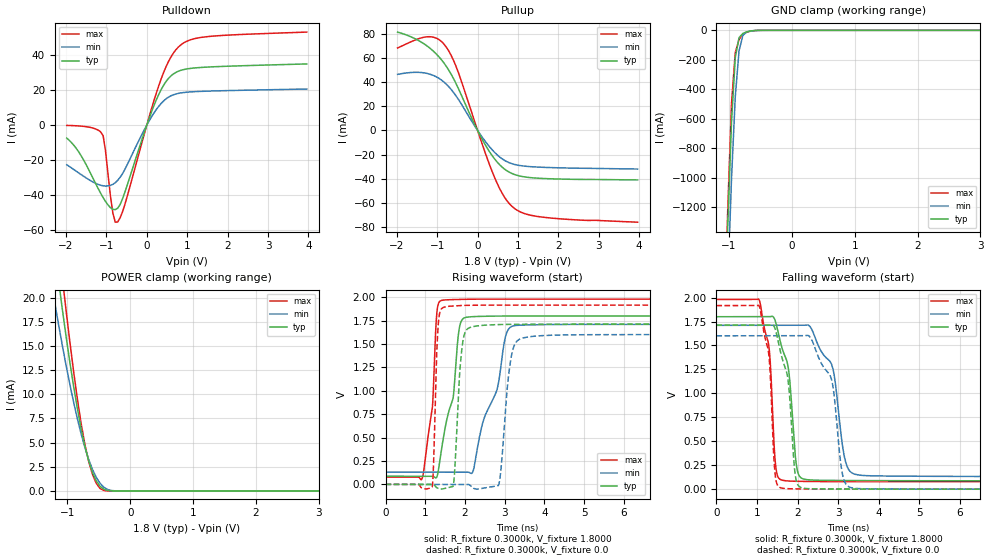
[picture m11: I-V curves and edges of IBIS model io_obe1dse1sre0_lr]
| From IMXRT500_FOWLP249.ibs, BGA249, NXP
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[Model] io_obe1dse1sre0_lr
|   Model io_obe1dse1sre0_lr
| Library cells for typ/min/max conditions are connected as defined below:
|  pad - External Pad
|  ipp_do - Core Input
|  ipp_obe - Output Buffer Enable
|  REFH3V3 - vdd1v8
|  gnde - gnde
|  ipp_dse - vdd
|  ipp_ina235_3v - NC
|  ipp_ina40_3v - NC
|  ipp_ina_mux - NC
|  ipp_ind - NC
|  ipp_ind_1p8v - NC
|  ipp_ind_3v - NC
|  vdd - vdd
|  vdd1v8 - vdd1v8
|  vdda - vdde3v3
|  vdde3v3 - vdde3v3
| All other pins connected to ground
Model_type I/O
Polarity   Non-Inverting
Enable   Active-High
Vinl =   0.5400V
Vinh =   1.2600V
Vmeas =  0.9000V
Cref =   25.0000pF
Rref =   0.5000k
Vref =   0.0V
C_comp   2.2672pF   2.1739pF   2.3940pF
[Temperature Range]   25.0000   0.1250k   -40.0000
[Voltage Range]   1.8000V   1.7100V   1.9800V
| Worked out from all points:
|   slope of the pulldown table from 0 to 0.27 V, typ, clamps not added: 16.6 ohm
|   slope of the pullup table from 0 to 0.27 V, typ, clamps not added: 16.6 ohm
|   GND clamp passes 1 mA (typ) near -0.57 V on its own axis
|   POWER clamp passes 1 mA (typ) near -0.54 V on its own axis
|   rising waveform, R_fixture 0.3000k, V_fixture 1.8000: 20-80 % time 372ps typ, 607ps min, 204ps max; typ from 0.087 V to 1.8 V
|   rising waveform, R_fixture 0.3000k, V_fixture 0.0: 20-80 % time 136ps typ, 195ps min, 81.2ps max; typ from 0 V to 1.71 V
|   falling waveform, R_fixture 0.3000k, V_fixture 1.8000: 20-80 % time 298ps typ, 454ps min, 191ps max; typ from 1.8 V to 0.087 V
|   falling waveform, R_fixture 0.3000k, V_fixture 0.0: 20-80 % time 282ps typ, 418ps min, 181ps max; typ from 1.71 V to 0 V
[Pulldown]
|Voltage   I(typ)   I(min)   I(max)
-1.98V    -7.47mA    -22.75mA   -160uA
-1.62V    -17.76mA   -28.49mA   -590uA
-1.08V    -41.65mA   -34.85mA   -6.067mA
-840mV    -48.37mA   -34.01mA   -50.49mA
-780mV    -48.54mA   -33.06mA   -55.75mA
-720mV    -47.69mA   -31.71mA   -55.6mA
-540mV    -38.38mA   -25.32mA   -45.39mA
240mV     14.74mA    9.107mA    18.7mA
540mV     26.9mA     16.1mA     36.66mA
780mV     30.94mA    18.23mA    44.81mA
1.44V     33.27mA    19.47mA    50.67mA
3.96V     35.14mA    20.73mA    53.44mA
[Pullup]
|Voltage   I(typ)   I(min)   I(max)
-1.98V    81.32mA    46.37mA    68.19mA
-1.2V     68.55mA    46.7mA     77.5mA
-960mV    61.01mA    43.15mA    75.21mA
-780mV    53.26mA    38.46mA    69.13mA
-480mV    34.98mA    25.95mA    48.25mA
-60mV     4.085mA    3.083mA    6.056mA
240mV     -14.69mA   -11.22mA   -23.31mA
600mV     -30.11mA   -23.3mA    -51.48mA
900mV     -36.25mA   -27.97mA   -64.14mA
1.2V      -38.57mA   -29.61mA   -69.11mA
1.68V     -39.78mA   -30.54mA   -71.94mA
3.96V     -40.89mA   -31.89mA   -75.83mA
[GND_clamp]
|Voltage   I(typ)   I(min)   I(max)
-1.98V    -17.54A    -17.55A    -18.13A
-1.08V    -2.178A    -2.567A    -2.121A
-1.02V    -1.334A    -1.74A     -1.223A
-960mV    -626.1mA   -1.012A    -499.4mA
-900mV    -186.7mA   -452.2mA   -152mA
-840mV    -49.63mA   -139.9mA   -62.86mA
-780mV    -21.48mA   -35.54mA   -26.58mA
-720mV    -10.4mA    -11.15mA   -13.18mA
-600mV    -1.573mA   -2.152mA   -2.249mA
-480mV    -123.2uA   -243.9uA   -63.17uA
3.96V     0A         0A         0A
[POWER_clamp]
|Voltage   I(typ)   I(min)   I(max)
-1.98V    72.06mA    51.35mA    77.71mA
-1.26V    28.12mA    21.78mA    33.04mA
-1.2V     24.9mA     19.47mA    29.3mA
-1.14V    21.8mA     17.23mA    25.64mA
-1.08V    18.82mA    15.06mA    22.09mA
-1.02V    15.98mA    12.99mA    18.67mA
-840mV    8.51mA     7.462mA    9.493mA
-720mV    4.608mA    4.475mA    4.783mA
-600mV    1.908mA    2.218mA    1.702mA
-540mV    1.04mA     1.402mA    786.7uA
-420mV    173.6uA    383.7uA    43.39uA
3.96V     0A         0A         0A
[Ramp]
| variable   typ   min   max
dV/dt_r  0.7875/0.2374n   0.6809/0.4047n   0.9809/0.1165n
dV/dt_f  0.7773/0.3694n   0.5489/0.6057n   0.9301/0.2312n
R_load = 50.0000
[Rising Waveform]
R_fixture= 0.3000k
V_fixture= 1.8000
V_fixture_min= 1.7100
V_fixture_max= 1.9800
|time   V(typ)   V(min)   V(max)
0s        87.2mV     130.7mV    78.02mV
929ps     87.2mV     130.7mV    74.45mV
1.183ns   87.73mV    130.7mV    843.2mV
1.286ns   76.21mV    130.7mV    1.81V
1.704ns   934.7mV    130.7mV    1.975V
1.872ns   1.699V     130.7mV    1.976V
2.226ns   1.793V     177.4mV    1.979V
3.087ns   1.799V     1.653V     1.98V
4.372ns   1.8V       1.708V     1.98V
500ns     1.8V       1.71V      1.98V
[Rising Waveform]
R_fixture= 0.3000k
V_fixture= 0.0
V_fixture_min= 0.0
V_fixture_max= 0.0
|time   V(typ)   V(min)   V(max)
0s        10.47nV    703.5nV    40.19nV
1.174ns   733.2uV    688.3nV    -24.45mV
1.342ns   -46.02mV   616.9nV    1.775V
1.698ns   -21.88mV   89.82nV    1.907V
1.953ns   1.545V     -10.26uV   1.911V
2.379ns   1.697V     -46.65mV   1.915V
2.857ns   1.708V     6.657mV    1.916V
3.283ns   1.71V      1.517V     1.916V
4.763ns   1.712V     1.598V     1.916V
500ns     1.712V     1.601V     1.916V
[Falling Waveform]
R_fixture= 0.3000k
V_fixture= 1.8000
V_fixture_min= 1.7100
V_fixture_max= 1.9800
|time   V(typ)   V(min)   V(max)
0s        1.8V       1.71V      1.98V
1.055ns   1.8V       1.71V      1.973V
1.301ns   1.8V       1.71V      1.458V
1.417ns   1.789V     1.71V      486.5mV
1.993ns   194.8mV    1.71V      81.82mV
2.286ns   97.01mV    1.706V     80.03mV
2.872ns   91.08mV    1.253V     78.75mV
3.245ns   90.04mV    213.8mV    78.4mV
4.379ns   88.45mV    136.2mV    78.08mV
500ns     87.2mV     130.7mV    78.02mV
[Falling Waveform]
R_fixture= 0.3000k
V_fixture= 0.0
V_fixture_min= 0.0
V_fixture_max= 0.0
|time   V(typ)   V(min)   V(max)
0s        1.712V     1.601V     1.916V
1.055ns   1.712V     1.601V     1.91V
1.296ns   1.712V     1.601V     1.383V
1.417ns   1.702V     1.601V     311.3mV
1.963ns   97.97mV    1.601V     2.595mV
2.257ns   5.203mV    1.605V     1.26mV
2.836ns   1.62mV     1.145V     440.4uV
3.158ns   1.207mV    76.9mV     248.9uV
3.9ns     660.4uV    2.672mV    74.97uV
500ns     364.7nV    1.163uV    271.1nV
